(* =======================================================================================================================================
   OOP: Extended sample
   =======================================================================================================================================
   Description: 
   This PLC sample contains an object-oriented program to control a sorting system.
   The application can be controlled via an integrated visualization.
   
   PLC_SortingSystem_PLC:
   The functionality of the sorting system is implemented within this PLC project (PLC_SortingSystem_PLC).
   It also contains the visualization to control the application.
   
   PLC_SortingSystem_Simu:
   To run the project without hardware, the simulation PLC can be used.
   For example, It simulates the cylinder positions and temperatures, as well as the sensor signals (correspondent to the box positions). 
   =======================================================================================================================================
   InfoSys:
   https://infosys.beckhoff.de/content/1033/tc3_sampleprogram1/45035996374683915.html?id=6126826020926170206
   https://infosys.beckhoff.de/content/1033/tc3_plc_intro/72057596565231755.html?id=3937754078542861062
   ======================================================================================================================================= *)
PROGRAM MAIN
VAR
	fbMachine				: FB_Machine;
	TaskInfo		  	 	: TaskInfo;	
	SystemInfo				: SystemInfo;
	EtherCAT				: FB_EcSlavesDiag;
	

END_VAR

// =========================================================

fbMachine();

// =========================================================

// Added

TaskInfo();

SystemInfo();

EtherCAT(MasterAmsNetId:= '' );

END_PROGRAM
